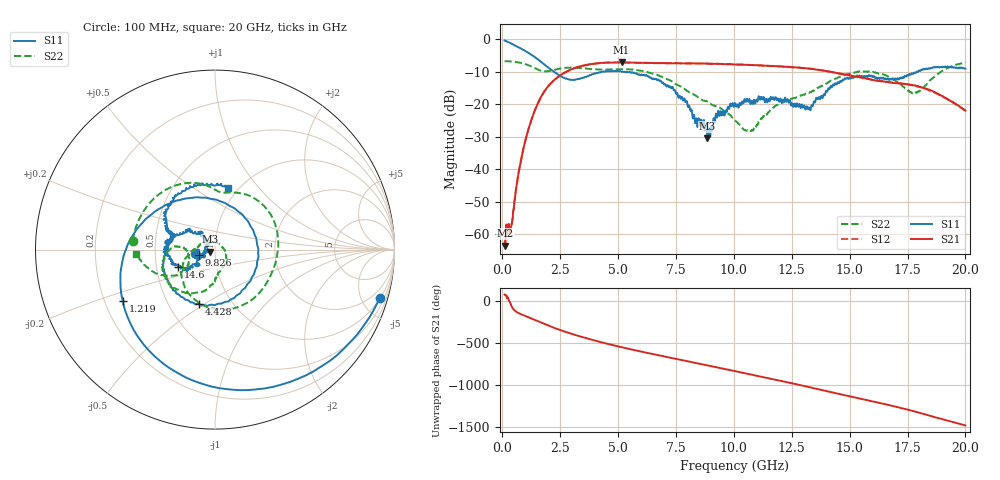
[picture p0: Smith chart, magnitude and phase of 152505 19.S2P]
!  2-Port S-parameters saved by WinCal
! VAR MeasName=S-Parameters (CALIBRATED_DATA) read from VNA (N5230C)
! VAR MeasDate=4/10/2015 9:30:11 AM
! VAR NAME=152505 19
! VAR FILENAME=152505 19.S2P
! VAR DATE=4/10/2015 9:30:11 AM
! VAR PHYS_PORTS=1,2
# Hz S DB R 50
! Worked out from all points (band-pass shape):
!   801 points, 100 MHz to 20 GHz, reference 50 ohm
!   highest |S21| = -7.13 dB at 5.15 GHz (marker M1); lowest = -63.5 dB at 124.9 MHz (marker M2)
!   |S21| within 3 dB of the highest: 2.732 GHz to 14.26 GHz (11.53 GHz wide, 136 % of centre)
!   lowest |S11| = -30.5 dB at 8.856 GHz (marker M3), VSWR 1.06, Z = 47.3 - j1.02 ohm
!   |S11| at or under -10 dB: 2.224 GHz to 4.344 GHz (2.119 GHz wide, 64.5 % of centre); 5.225 GHz to 5.287 GHz (61.71 MHz wide, 1.17 % of centre); 5.306 GHz to 17.88 GHz (12.58 GHz wide, 108 % of centre)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
!   |S22| runs from -28.3 to -6.8 dB; largest |S21 - S12| = 0.0068
!   S11 on the Smith chart (normalised r, x): 100 MHz: 1.05, -6.80; 1.219 GHz: 0.27, -0.24; 4.428 GHz: 0.71, -0.48; 9.826 GHz: 0.83, -0.05; 14.6 GHz: 0.65, -0.13; 20 GHz: 0.89, +0.70
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1e8  -0.38 -16.4  -62.58 72.7  -63.67 80.5  -6.75 173.9
1.24875e8  -0.46 -20.0  -63.47 63.5  -62.07 58.9  -6.75 172.3
3.985e8  -1.36 -57.5  -57.14 -64.4  -57.18 -65.4  -6.86 155.3
5.975e8  -2.07 -82.4  -45.93 -129.9  -45.92 -129.8  -7.02 143.0
1.219375e9  -4.60 -150.7  -25.64 153.3  -25.60 153.3  -8.26 106.1
2.1895e9  -9.79 118.0  -12.90 43.1  -12.91 42.9  -9.55 72.5
3.43325e9  -12.00 -27.2  -8.22 -69.0  -8.23 -68.9  -8.92 13.0
4.42825e9  -10.00 -105.9  -7.22 -142.8  -7.21 -142.9  -9.35 -27.2
5.149625e9  -10.03 -142.1  -7.13 169.2  -7.16 169.1  -9.21 -56.2
6.741625e9  -12.37 160.1  -7.36 74.2  -7.34 73.8  -11.09 -124.9
7.81125e9  -18.88 129.9  -7.44 13.3  -7.42 13.6  -14.98 -161.8
8.856e9  -30.53 -158.7  -7.51 -46.4  -7.53 -46.2  -19.25 174.8
9.826125e9  -20.36 -161.1  -7.69 -101.4  -7.65 -101.5  -23.27 144.3
1.005e10  -19.61 -154.2  -7.75 -114.4  -7.75 -114.5  -24.84 125.3
1.07465e10  -19.49 -163.3  -7.94 -154.3  -7.92 -154.2  -28.28 41.9
1.146788e10  -18.81 -173.3  -8.17 163.8  -8.13 163.8  -22.63 -31.6
1.246288e10  -20.26 -170.2  -8.53 104.7  -8.63 104.5  -18.34 -74.3
1.338325e10  -20.48 -150.5  -9.17 48.3  -9.14 48.3  -15.92 -88.5
1.460212e10  -12.80 -154.7  -10.67 -27.4  -10.57 -28.1  -11.51 -115.0
1.669162e10  -12.46 163.2  -13.20 -155.4  -13.25 -156.3  -11.63 -177.6
1.7811e10  -10.35 155.1  -14.26 128.0  -14.34 126.5  -16.63 -167.1
2e10  -9.05 78.2  -21.96 -37.3  -22.00 -36.4  -7.12 -177.0
